PROGRAM MAIN
VAR
    FB_FileOpen:                FB_FileOpen;//创建txt文件（utf8格式）
	FB_FileWrite:               FB_FileWrite;//写入数据到txt文档里
	FB_FileClose:               FB_FileClose;//关闭txt文件
	b_open:                     BOOL;//Fileopen触发位
	b_write:                    BOOL;//FileWrite触发位
	b_close:                    BOOL;//FileClose触发位
    wstring1:                   WSTRING := "倍福中国$R";//需写入的中文字符
	{attribute 'TcEncoding':='UTF-8'}
	wstring2:                   STRING;	//用于转码后的字符
    step:                       INT;//Case步
	Ton1:                       TON;//定时器
	b_on1:                      BOOL;//定时器触发位
	Wlen_test:                  INT;//以int变量的形式表示测算出的字符长度（可根据写入的字符数量更改数据类型）
END_VAR

WSTRING_TO_UTF8(pDstUTF8:=ADR(wstring2) , pSrcWSTRING:=ADR(wstring1) , nDstSize:=SIZEOF(wstring2) );//Wstring转UTF8
Wlen_test:=WLEN(wstring1);//用wlen计算中文字符数量


file_fb();
CASE step OF
0:
b_open:=TRUE;
b_on1:=TRUE;
IF b_open=TRUE AND Ton1.Q THEN
   b_open:=FALSE;
   b_on1:=FALSE;
   step:=10;
END_IF

10:
b_write:=TRUE;
b_on1:=TRUE;
IF b_write=TRUE AND Ton1.Q THEN
   b_write:=FALSE;
   b_on1:=FALSE;
   step:=20;
END_IF

20:
b_close:=TRUE;
b_on1:=TRUE;
IF b_close=TRUE AND Ton1.Q THEN
   b_close:=FALSE;
   b_on1:=FALSE;
   step:=0;
END_IF
END_CASE

ACTION file_fb:
FB_FileOpen( 
	sPathName:='E:\TESTFILE1.txt' , //目标txt路径和文件名
	nMode:=FOPEN_MODEAPPEND OR FOPEN_MODEPLUS OR FOPEN_MODETEXT,//写入模式
	ePath:=1 , //根据路径选择打开模式
	bExecute:=b_open , 
	tTimeout:=T#3S , 
 );
 
 FB_FileWrite( 
	hFile:=FB_FileOpen.hFile,
	pWriteBuff:=ADR(wstring2),
	cbWriteLen:=3*wlen_test-2,//在UTF-8格式中中文字符占三个字节长度
	bExecute:=b_write , 
	tTimeout:=T#3S
 );
 
FB_FileClose( 
	hFile:=FB_FileOpen.hFile , 
	bExecute:=b_close,
	tTimeout:=T#3S,
);


Ton1(IN:=b_on1 , PT:=T#3S , Q=> , ET=> );
END_ACTION

END_PROGRAM
